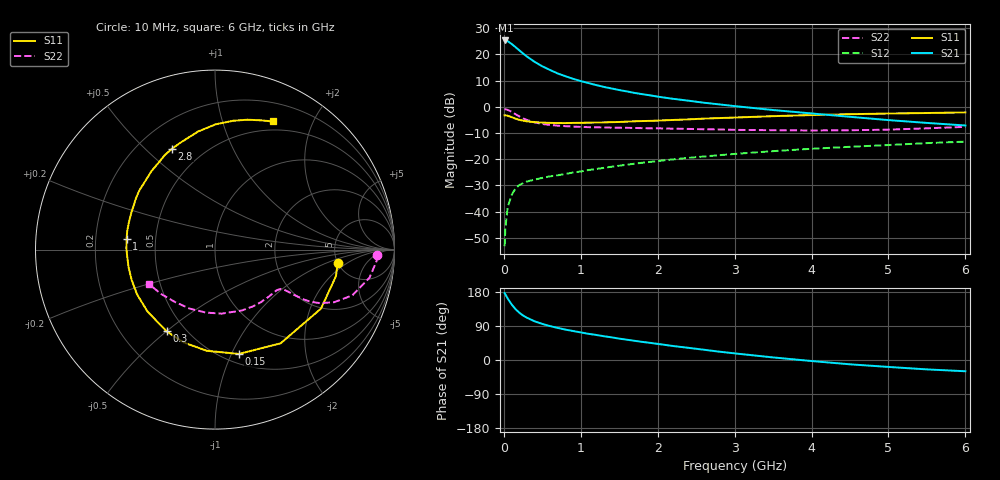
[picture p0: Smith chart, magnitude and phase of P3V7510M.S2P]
! SIEMENS Small Signal Semiconductors
! BFP181
! Si NPN RF Bipolar Junction Transistor in SOT143
! VCE = 0.75 V  IC = 10 mA
! Common Emitter S-Parameters:  March  1996
# GHz  S  MA  R  50
!  f  S11  S21  S12  S22
! GHz  MAG  ANG  MAG  ANG  MAG  ANG  MAG  ANG
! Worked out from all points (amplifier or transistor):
!   36 points, 10 MHz to 6 GHz, reference 50 ohm
!   highest |S21| = 25.3 dB at 20 MHz (marker M1)
!   |S21| within 3 dB of that: start of sweep to 170.3 MHz
!   unconditionally stable (mu >= 1): start of sweep to 12.05 MHz; 454.8 MHz to end of sweep
!   at 250 MHz: K = 0.63, MSG = 24.7 dB, |S12| = -29.1 dB
!   at 1.4 GHz: K = 1.80, MAG = 9.8 dB, |S12| = -22.8 dB
!   at 6 GHz: K = 1.62, MAG = -1.5 dB, |S12| = -13.3 dB
!   S11 on the Smith chart (normalised r, x): 10 MHz: 5.01, -1.39; 150 MHz: 0.59, -1.07; 300 MHz: 0.40, -0.50; 1 GHz: 0.34, +0.05; 2.8 GHz: 0.34, +0.61; 6 GHz: 0.40, +1.47
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0.01  0.6878 -6.1  18.45 176.5  0.0022 84.2  0.9032 -2.0
0.02  0.69 -12.4  18.48 173.2  0.0049 80.2  0.9024 -4.1
0.05  0.6758 -29.1  17.86 162.3  0.0122 77.2  0.8751 -10.3
0.1  0.6375 -55.0  15.9 147.1  0.0207 62.9  0.8069 -18.4
0.15  0.5964 -77.1  13.87 134.5  0.0276 55.2  0.726 -23.8
0.2  0.5656 -94.7  12.02 125.0  0.0323 49.8  0.6577 -27.0
0.25  0.5461 -108.7  10.4 117.4  0.035 45.4  0.6037 -28.7
0.3  0.5293 -120.6  9.126 111.6  0.0376 43.7  0.5626 -29.4
0.4  0.5102 -137.5  7.226 102.0  0.041 40.7  0.5058 -29.8
0.5  0.501 -150.2  5.931 95.2  0.0441 39.9  0.4717 -29.9
0.6  0.4942 -160.1  5.056 89.5  0.0472 40.6  0.4519 -30.1
0.7  0.4916 -168.2  4.335 84.7  0.0495 41.4  0.4383 -30.4
0.8  0.4906 -175.4  3.844 80.2  0.0526 42.0  0.428 -30.9
1  0.4959 173.1  3.103 72.8  0.0585 43.4  0.4146 -32.8
1.1  0.4998 168.2  2.841 69.1  0.0623 43.8  0.4101 -33.9
1.5  0.5146 151.7  2.092 56.4  0.0754 45.0  0.3999 -39.6
2.2  0.5623 129.1  1.424 36.9  0.0996 43.3  0.3838 -52.7
2.8  0.6108 113.0  1.115 22.0  0.1197 39.9  0.3711 -66.0
3.5  0.6647 98.1  0.87 6.8  0.143 35.3  0.3586 -84.2
4.5  0.7248 82.0  0.646 -11.4  0.173 27.1  0.3578 -113.2
5.5  0.7633 70.7  0.494 -24.8  0.2036 19.3  0.3894 -140.6
6  0.7834 65.7  0.441 -29.7  0.2169 14.8  0.4159 -152.8
